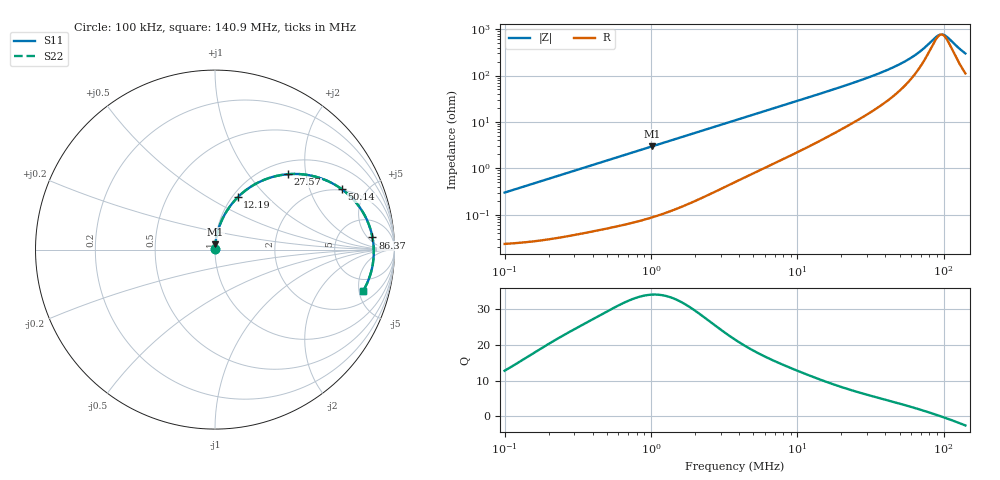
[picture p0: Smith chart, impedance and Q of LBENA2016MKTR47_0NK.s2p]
! LBENA2016MKTR47_0NK  S-PARAMETER MODEL  ( General Type )
! Model Generated by TAIYO YUDEN Corporation (http://www.ty-top.com)
! Version 1.0
! TAIYO YUDEN Control No. 211203
! Copyright(c) 2021 TAIYO YUDEN CO.,LTD. All Rights Reserved.
! Product Description (link to TY-COMPAS)
! https://ds.yuden.co.jp/TYCOMPAS/or/detail?pn=LBENA2016MKTR47M0NK&u=M
! Products Name : Inductors
! Characteristics :
!  Inductance : 0.47 uH , SRF(min) : -Hz , DC Resistance(max) : 0.025 Ohm
!  Rated Current : Saturation :4800 mA , Temp Rise : 4700 mA
!  Case Size : 2.0 x 1.6 / 0.079 x 0.063 [mm/inch] , Thickness : 1.2 / 0.047 [mm/inch]
!  (Conditions: Temperature = 25 degC , DC Bias Current/Voltage = 0A / 0V)
! External Node Assignments :
!  1  o---GGG---o  2
! GND o---------o GND
! Frequency Range : 0.1MHz  -  140.89697MHz  [ 402 STEP ]
# MHz S RI R 50
! Freq[MHz].  S11 Real  S11 Imag  S21 Real  S21 Imag  S12 Real  S12 Imag  S22 Real  S22 Imag
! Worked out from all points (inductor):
!   401 points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, 100 kHz to 140.9 MHz, reference 50 ohm
!   read as one part in series: L = 476 nH near 103.7 kHz
!   highest Q = 34 at 1.018 MHz (marker M1), where L = 465 nH
!   self-resonance near 96.42 MHz
!   S11 on the Smith chart (normalised r, x): 100 kHz: 1.00, +0.01; 12.19 MHz: 1.06, +0.69; 27.57 MHz: 1.25, +1.59; 50.14 MHz: 1.95, +3.38; 86.37 MHz: 11, +7; 140.9 MHz: 3.22, -5.55
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0.1  0.000244 0.00299  0.9998 -0.00299  0.9998 -0.00299  0.000244 0.00299
0.336853  0.000491 0.00996  0.9995 -0.00996  0.9995 -0.00996  0.000491 0.00996
1.017767  0.00176 0.0297  0.9982 -0.0297  0.9982 -0.0297  0.00176 0.0297
1.134703  0.00207 0.033  0.9979 -0.033  0.9979 -0.033  0.00207 0.033
3.753625  0.0164 0.1057  0.9836 -0.1057  0.9836 -0.1057  0.0164 0.1057
7.340476  0.0536 0.1945  0.9464 -0.1945  0.9464 -0.1945  0.0536 0.1945
12.19403  0.1266 0.2914  0.8734 -0.2914  0.8734 -0.2914  0.1266 0.2914
12.64421  0.1343 0.2989  0.8657 -0.2989  0.8657 -0.2989  0.1343 0.2989
18.5016  0.2415 0.3742  0.7585 -0.3742  0.7585 -0.3742  0.2415 0.3742
27.56759  0.4078 0.4203  0.5922 -0.4203  0.5922 -0.4203  0.4078 0.4203
34.26619  0.516 0.4157  0.484 -0.4157  0.484 -0.4157  0.516 0.4157
42.59248  0.6275 0.3823  0.3725 -0.3823  0.3725 -0.3823  0.6275 0.3823
50.13987  0.707 0.3362  0.293 -0.3362  0.293 -0.3362  0.707 0.3362
57.96438  0.77 0.2803  0.23 -0.2803  0.23 -0.2803  0.77 0.2803
67.00994  0.822 0.2115  0.178 -0.2115  0.178 -0.2115  0.822 0.2115
74.70897  0.8519 0.1529  0.1481 -0.1529  0.1481 -0.1529  0.8519 0.1529
86.36759  0.8773 0.0678  0.1227 -0.0678  0.1227 -0.0678  0.8773 0.0678
94.561  0.8841 0.0121  0.1159 -0.0121  0.1159 -0.0121  0.8841 0.0121
101.6719  0.8843 -0.0331  0.1157 0.0331  0.1157 0.0331  0.8843 -0.0331
107.3539  0.8813 -0.067  0.1187 0.067  0.1187 0.067  0.8813 -0.067
131.0426  0.8473 -0.1876  0.1527 0.1876  0.1527 0.1876  0.8473 -0.1876
140.897  0.8264 -0.2284  0.1736 0.2284  0.1736 0.2284  0.8264 -0.2284
